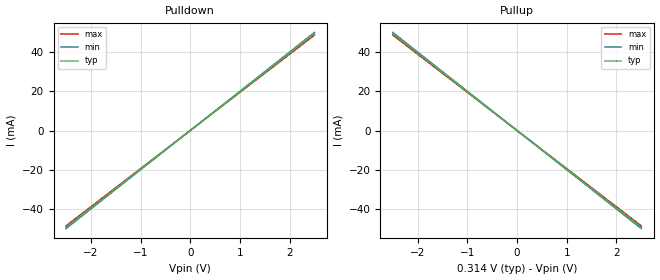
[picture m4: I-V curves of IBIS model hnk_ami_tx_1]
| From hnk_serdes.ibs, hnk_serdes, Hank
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|   model   hnk_ami_tx_1
[Model] hnk_ami_tx_1
Model_type Output
C_comp 800f 750f 850f
Cref = 0
[Model Spec]
Vmeas .157 .15 .165
Vref .157 .15 .165
[Temperature Range]  25 100 0
[Voltage Range] .314 .299 .329
[Algorithmic Model]
Executable Windows_VisualStudio7.1.3088_64 hnkffe.dll hnkffe.ami
Executable Linux_gcc3.2.3_64 hnkffe.linux.so hnkffe.ami
[End Algorithmic Model]
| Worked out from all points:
|   slope of the pulldown table from 0 to 0.047 V, typ, clamps not added: 50.4 ohm
|   slope of the pullup table from 0 to 0.047 V, typ, clamps not added: 50.4 ohm
[Pulldown]
-2.5V     -49.56mA   -50.28mA   -48.88mA
0V        0A         0A         0A
2.5V      49.56mA    50.28mA    48.88mA
[Pullup]
-2.5V     49.56mA    50.28mA    48.88mA
0V        0A         0A         0A
2.5V      -49.56mA   -50.28mA   -48.88mA
[Ramp]
dV/dt_r .094/60f .09/60f .098/60f
dV/dt_f .094/60f .09/60f .098/60f
